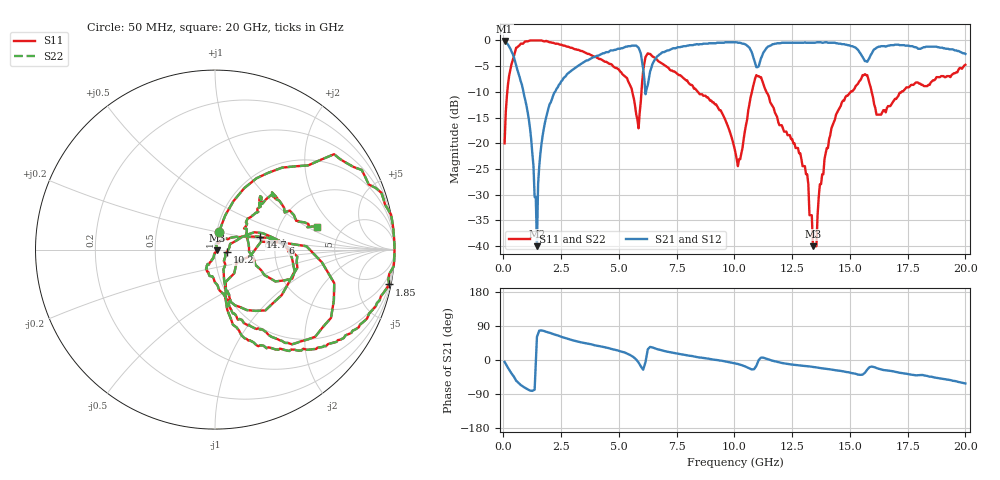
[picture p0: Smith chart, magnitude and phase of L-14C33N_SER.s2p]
# MHZ S MA R 50
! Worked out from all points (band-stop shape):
!   400 points, 50 MHz to 20 GHz, reference 50 ohm
!   highest |S21| = -0.09 dB at 50 MHz (marker M1); lowest = -40.0 dB at 1.45 GHz (marker M2)
!   |S21| within 3 dB of the highest: 6.654 GHz to 10.81 GHz (4.153 GHz wide, 47.6 % of centre); 11.19 GHz to 15.53 GHz (4.343 GHz wide, 32.5 % of centre)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
!   lowest |S11| = -40.0 dB at 13.4 GHz (marker M3), VSWR 1.02, Z = 50.9 - j0.403 ohm
!   |S11| at or under -10 dB: 8.419 GHz to 10.76 GHz (2.34 GHz wide, 24.4 % of centre); 11.38 GHz to 15.03 GHz (3.647 GHz wide, 27.6 % of centre); 15.94 GHz to 17.23 GHz (1.29 GHz wide, 7.77 % of centre)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
!   |S22| runs from -40.0 to 0.0 dB; largest |S21 - S12| = 0
!   S11 on the Smith chart (normalised r, x): 50 MHz: 1.02, +0.20; 1.85 GHz: 1, -10; 6 GHz: 2.20, +0.20; 10.2 GHz: 1.15, -0.04; 14.7 GHz: 1.64, +0.25; 20 GHz: 3.25, +1.23
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50  0.1 77.5  0.99 -4.9  0.99 -4.9  0.1 77.5
350  0.59 50.7  0.78 -35.5  0.78 -35.5  0.59 50.7
1100  0.99 13.0  0.17 -79.1  0.17 -79.1  0.99 13.0
1400  1 2.9  0.03 -8.6  0.03 -8.6  1 2.9
1450  1 1.6  0.01 61.0  0.01 61.0  1 1.6
1550  1 -2.1  0.06 77.7  0.06 77.7  1 -2.1
1850  0.99 -11.3  0.18 74.4  0.18 74.4  0.99 -11.3
3400  0.79 -44.5  0.6 46.1  0.6 46.1  0.79 -44.5
5350  0.43 -76.6  0.87 16.8  0.87 16.8  0.43 -76.6
5850  0.14 -30.3  0.85 -6.7  0.85 -6.7  0.14 -30.3
6000  0.38 5.9  0.63 -21.3  0.63 -21.3  0.38 5.9
6150  0.69 -15.7  0.3 -5.4  0.3 -5.4  0.69 -15.7
6700  0.63 -53.8  0.71 28.1  0.71 28.1  0.63 -53.8
10050  0.08 -51.6  0.96 -9.2  0.96 -9.2  0.08 -51.6
10200  0.07 -12.7  0.95 -11.4  0.95 -11.4  0.07 -12.7
11150  0.44 -50.3  0.67 6.4  0.67 6.4  0.44 -50.3
13350  0.02 -87.9  0.95 -17.9  0.95 -17.9  0.02 -87.9
13400  0.01 -23.3  0.95 -18.3  0.95 -18.3  0.01 -23.3
13950  0.08 47.5  0.96 -23.0  0.96 -23.0  0.08 47.5
14700  0.26 15.8  0.92 -29.8  0.92 -29.8  0.26 15.8
16700  0.23 40.3  0.89 -28.3  0.89 -28.3  0.23 40.3
20000  0.58 12.5  0.74 -62.0  0.74 -62.0  0.58 12.5
